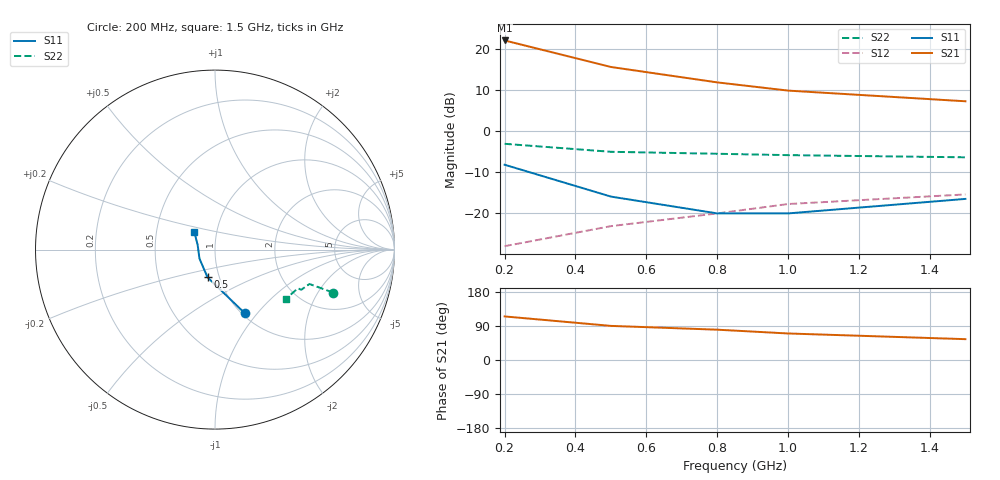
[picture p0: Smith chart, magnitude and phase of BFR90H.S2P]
!  BFR90H.S2P
!  BFR90
!  VCE=10V; IC=10mA
#  GHZ S MA R 50
!  S-PARAMETER DATA
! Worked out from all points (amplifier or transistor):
!   5 points, 200 MHz to 1.5 GHz, reference 50 ohm
!   highest |S21| = 22.0 dB at 200 MHz (marker M1)
!   |S21| within 3 dB of that: start of sweep to 339.7 MHz
!   unconditionally stable (mu >= 1): 565.1 MHz to end of sweep
!   at 200 MHz: K = 0.70, MSG = 25.0 dB, |S12| = -28.0 dB
!   at 800 MHz: K = 1.06, MAG = 14.4 dB, |S12| = -20.0 dB
!   at 1.5 GHz: K = 1.09, MAG = 9.5 dB, |S12| = -15.4 dB
!   S11 on the Smith chart (normalised r, x): 200 MHz: 1.03, -0.86; 500 MHz: 0.88, -0.28; 1.5 GHz: 0.78, +0.15
0.2  0.39 -65.0  12.6 115.0  0.04 65.0  0.7 -20.0
0.5  0.16 -105.0  6 90.0  0.07 70.0  0.56 -20.0
0.8  0.1 -150.0  3.9 80.0  0.1 70.0  0.53 -25.0
1  0.1 165.0  3.1 70.0  0.13 70.0  0.51 -25.0
1.5  0.15 140.0  2.3 55.0  0.17 70.0  0.48 -35.0
